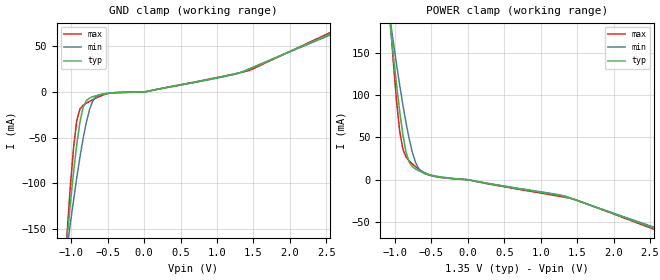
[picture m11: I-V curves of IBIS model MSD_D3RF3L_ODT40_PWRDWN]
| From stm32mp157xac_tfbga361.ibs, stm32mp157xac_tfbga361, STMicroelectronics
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[Model] MSD_D3RF3L_ODT40_PWRDWN
Model_type   Input
C_comp 2.509pF   2.467pF   2.564pF
Vinh = 810.000mV
Vinl = 540.000mV
[Model Spec]
Vinh   810.000mV   777.000mV   860.000mV
Vinl   540.000mV   507.000mV   590.000mV
[Temperature Range]   25.000   125.000   -40.000
[Voltage Range]   1.350V   1.283V   1.450V
[GND Clamp Reference]   0.00V   0.00V   0.00V
[POWER Clamp Reference]   1.350V   1.283V   1.450V
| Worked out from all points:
|   GND clamp passes 1 mA (typ) near -0.45 V on its own axis
|   POWER clamp passes 1 mA (typ) near -0.15 V on its own axis
[GND Clamp]
-1.318V   -417.1mA   -342.8mA   -535.6mA
-1.055V   -160.4mA   -171.5mA   -154.9mA
-1.011V   -122.8mA   -144.6mA   -104.1mA
-966.7mV  -88.16mA   -118.8mA   -61.12mA
-922.7mV  -57.63mA   -94.23mA   -31.44mA
-834.9mV  -16.71mA   -50.78mA   -14.6mA
-747mV    -6.626mA   -19.06mA   -10.27mA
-659.1mV  -4.14mA    -5.18mA    -6.61mA
-571.2mV  -2.434mA   -2.258mA   -3.598mA
200nV     3.413nA    3.285nA    3.464nA
1.45V     25.37mA    25.7mA     23.83mA
2.68V     68.1mA     66.81mA    69.97mA
[Power Clamp]
-1.33V    442.7mA    365.2mA    568.3mA
-1.067V   186.3mA    191.4mA    194mA
-1.023V   149mA      164.1mA    141.7mA
-978.8mV  113.9mA    137.7mA    94.8mA
-934.9mV  81.74mA    112.7mA    57.95mA
-890.9mV  53.76mA    89.11mA    36.38mA
-803mV    20.55mA    48.25mA    22.19mA
-715.1mV  12.58mA    20.14mA    15.35mA
-627.3mV  8.939mA    8.723mA    9.956mA
-495.5mV  5.328mA    4.647mA    4.764mA
1.35V     -19.96mA   -20.38mA   -21.21mA
2.668V    -61.12mA   -59.8mA    -62.59mA
